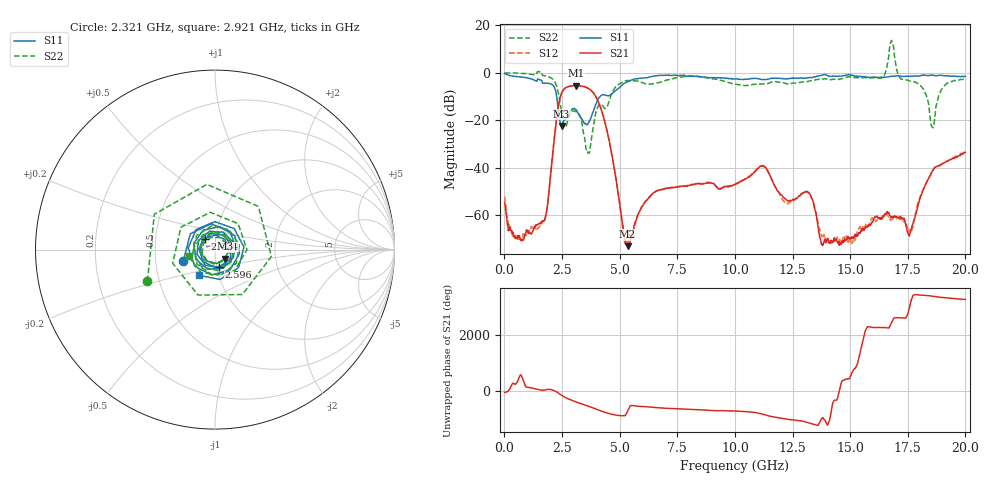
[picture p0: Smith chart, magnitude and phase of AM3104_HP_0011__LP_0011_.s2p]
!Created with skrf (http://scikit-rf.org).
# Hz S RI R 50.0
!freq ReS11 ImS11 ReS21 ImS21 ReS12 ImS12 ReS22 ImS22
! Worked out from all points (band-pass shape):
!   1601 points, 10 MHz to 20 GHz, reference 50 ohm
!   highest |S21| = -5.32 dB at 3.108 GHz (marker M1); lowest = -73.0 dB at 5.345 GHz (marker M2)
!   |S21| within 3 dB of the highest: 2.489 GHz to 3.853 GHz (1.364 GHz wide, 43 % of centre)
!   lowest |S11| = -22.3 dB at 2.484 GHz (marker M3), VSWR 1.17, Z = 55.9 - j5.62 ohm
!   |S11| at or under -10 dB: 2.269 GHz to 4.146 GHz (1.877 GHz wide, 58.5 % of centre)
!   |S22| runs from -33.9 to 13.7 dB; largest |S21 - S12| = 0.03
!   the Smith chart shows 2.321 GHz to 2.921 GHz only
!   S11 on the Smith chart (normalised r, x): 2.321 GHz: 0.70, -0.09; 2.434 GHz: 0.88, +0.11; 2.596 GHz: 1.03, -0.20; 2.921 GHz: 0.80, -0.24
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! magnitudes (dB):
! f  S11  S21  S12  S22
! 10 MHz  -0.3  -54.6  -52.1  0.0
! 447.3 MHz  -1.5  -69.2  -69.7  -0.1
! 1.697 GHz  -4.4  -62.4  -62.5  -1.1
! 2.321 GHz  -14.6  -15.3  -15.3  -7.6
! 2.434 GHz  -21.5  -9.8  -9.9  -13.6
! 2.484 GHz  -22.3  -8.4  -8.5  -16.8
! 2.596 GHz  -19.9  -6.8  -6.7  -22.3
! 2.921 GHz  -15.4  -5.5  -5.6  -16.4
! 3.108 GHz  -15.6  -5.3  -5.3  -16.4
! 3.346 GHz  -19.4  -5.5  -5.6  -20.2
! 3.633 GHz  -21.3  -6.5  -6.6  -33.4
! 4.283 GHz  -9.2  -18.0  -17.9  -14.1
! 5.345 GHz  -3.8  -73.0  -71.0  -3.2
! 6.682 GHz  -1.1  -49.5  -49.4  -4.2
! 10.01 GHz  -2.6  -47.1  -47.1  -4.8
! 11.2 GHz  -2.8  -39.1  -39.3  -4.6
! 13.34 GHz  -2.0  -52.8  -52.9  -3.3
! 13.84 GHz  -0.8  -71.9  -68.3  -2.6
! 16.68 GHz  -1.6  -59.1  -60.6  7.2
! 17.58 GHz  -1.4  -68.7  -66.8  -3.4
! 18.58 GHz  -0.9  -41.1  -41.5  -23.0
! 20 GHz  -1.4  -33.5  -33.2  -2.5
